FUNCTION_BLOCK p12_controlLight
VAR_INPUT
	button: BOOL;
END_VAR
VAR_OUTPUT
	light: BOOL;
END_VAR
VAR
	positiveEdgeDetection: R_TRIG;
	buttonPulse: BOOL;
	memoryCell: SR;
END_VAR

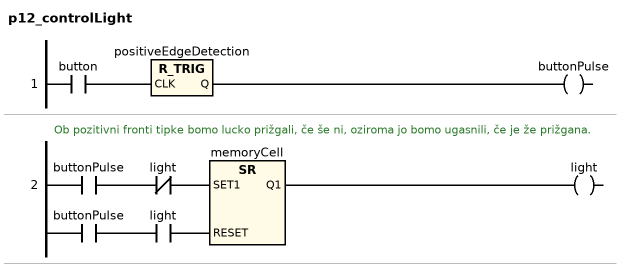
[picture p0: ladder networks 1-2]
// NETWORK 1
positiveEdgeDetection(CLK := button); // R_TRIG
buttonPulse := positiveEdgeDetection.Q;

// NETWORK 2
// Ob pozitivni fronti tipke bomo lucko prižgali, če še ni, oziroma jo bomo ugasnili, če je že prižgana.
memoryCell(SET1 := buttonPulse AND NOT light, RESET := buttonPulse AND light); // SR
light := memoryCell.Q1;

END_FUNCTION_BLOCK
